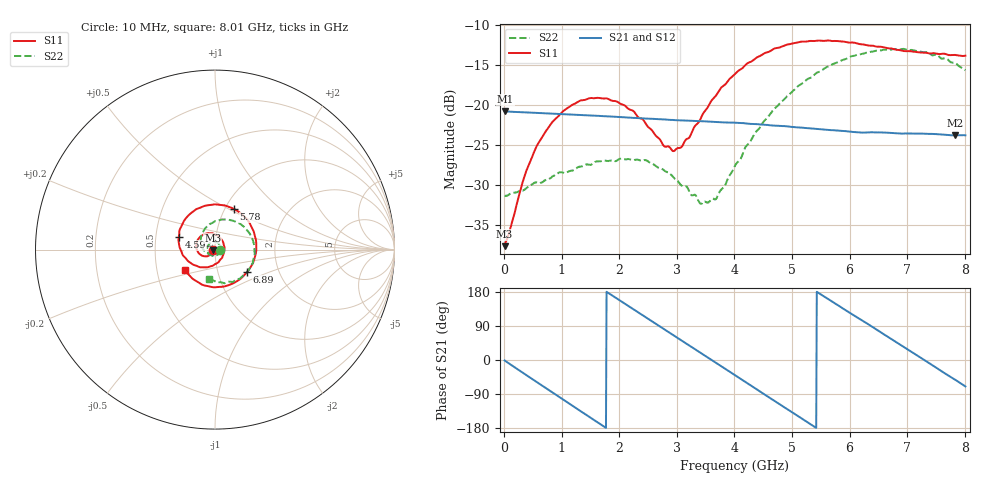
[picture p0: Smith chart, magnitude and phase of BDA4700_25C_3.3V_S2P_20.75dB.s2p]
!Agilent Technologies,E5071B,MY42404982,A.09.10
!Date: Mon Oct 20 18:11:46 2025
!Data & Calibration Information:
!Freq	S11:SOLT2(ON)	S21:SOLT2(ON)	S12:SOLT2(ON)	S22:SOLT2(ON)
# Hz S RI R 50
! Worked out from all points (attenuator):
!   801 points, 10 MHz to 8.01 GHz, reference 50 ohm
!   highest |S21| = -20.83 dB at 20 MHz (marker M1); lowest = -23.8 dB at 7.83 GHz (marker M2)
!   lowest |S11| = -37.7 dB at 10 MHz (marker M3), VSWR 1.03, Z = 48.7 - j0.147 ohm
!   |S11| at or under -10 dB: start of sweep to end of sweep
!   |S22| runs from -32.4 to -13.0 dB; largest |S21 - S12| = 0.0011
!   S11 on the Smith chart (normalised r, x): 10 MHz: 0.97, -0.00; 4.59 GHz: 0.66, +0.10; 5.78 GHz: 1.10, +0.53; 6.89 GHz: 1.38, -0.36; 8.01 GHz: 0.70, -0.17
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1e7  -0.013 -0.00151  0.0909 -0.00195  0.0909 -0.00202  0.0269 -0.000791
2e7  -0.0133 -0.00232  0.0908 -0.00349  0.0908 -0.00377  0.0268 -0.00108
3.5e8  -0.0235 -0.0262  0.0724 -0.0528  0.0723 -0.0528  0.0228 -0.0183
5.8e8  -0.0422 -0.0371  0.0452 -0.0765  0.0452 -0.0765  0.0145 -0.0292
1e9  -0.0858 -0.0245  -0.0179 -0.0856  -0.0178 -0.0857  -0.0147 -0.0348
1.35e9  -0.1056 0.015  -0.0631 -0.0588  -0.0631 -0.0589  -0.0369 -0.0181
1.97e9  -0.0566 0.0874  -0.0793 0.0273  -0.0793 0.0274  -0.0346 0.0287
2.68e9  0.0448 0.043  -0.001 0.0812  -0.00118 0.0812  0.0139 0.0379
2.93e9  0.0513 -0.00208  0.0324 0.0734  0.0324 0.0733  0.0257 0.0245
3.06e9  0.0467 -0.0267  0.0478 0.064  0.0472 0.0643  0.0283 0.0145
3.43e9  -0.00376 -0.0843  0.0754 0.0232  0.0754 0.0232  0.0196 -0.0138
3.69e9  -0.0608 -0.098  0.0771 -0.0114  0.0771 -0.0117  0.000707 -0.026
4.01e9  -0.1369 -0.074  0.059 -0.0496  0.0591 -0.0495  -0.0321 -0.0262
4.59e9  -0.2013 0.0716  -0.00985 -0.0739  -0.00968 -0.074  -0.078 0.033
5.35e9  -0.0441 0.2464  -0.0703 -0.00953  -0.0703 -0.00998  -0.0156 0.1482
5.78e9  0.1063 0.2266  -0.0573 0.0385  -0.057 0.0384  0.0797 0.1653
6.24e9  0.2147 0.1028  -0.0145 0.0653  -0.0134 0.0656  0.1797 0.1068
6.68e9  0.2178 -0.0571  0.0338 0.0574  0.0339 0.0575  0.22 -0.00163
6.89e9  0.18 -0.1242  0.0509 0.0419  0.0512 0.0416  0.2133 -0.0618
7.34e9  0.0401 -0.207  0.0656 -0.00496  0.0657 -0.00492  0.141 -0.1603
7.83e9  -0.126 -0.1614  0.0397 -0.0506  0.0396 -0.0507  0.0114 -0.182
8.01e9  -0.1669 -0.1147  0.0223 -0.0604  0.0225 -0.0603  -0.0317 -0.1611
